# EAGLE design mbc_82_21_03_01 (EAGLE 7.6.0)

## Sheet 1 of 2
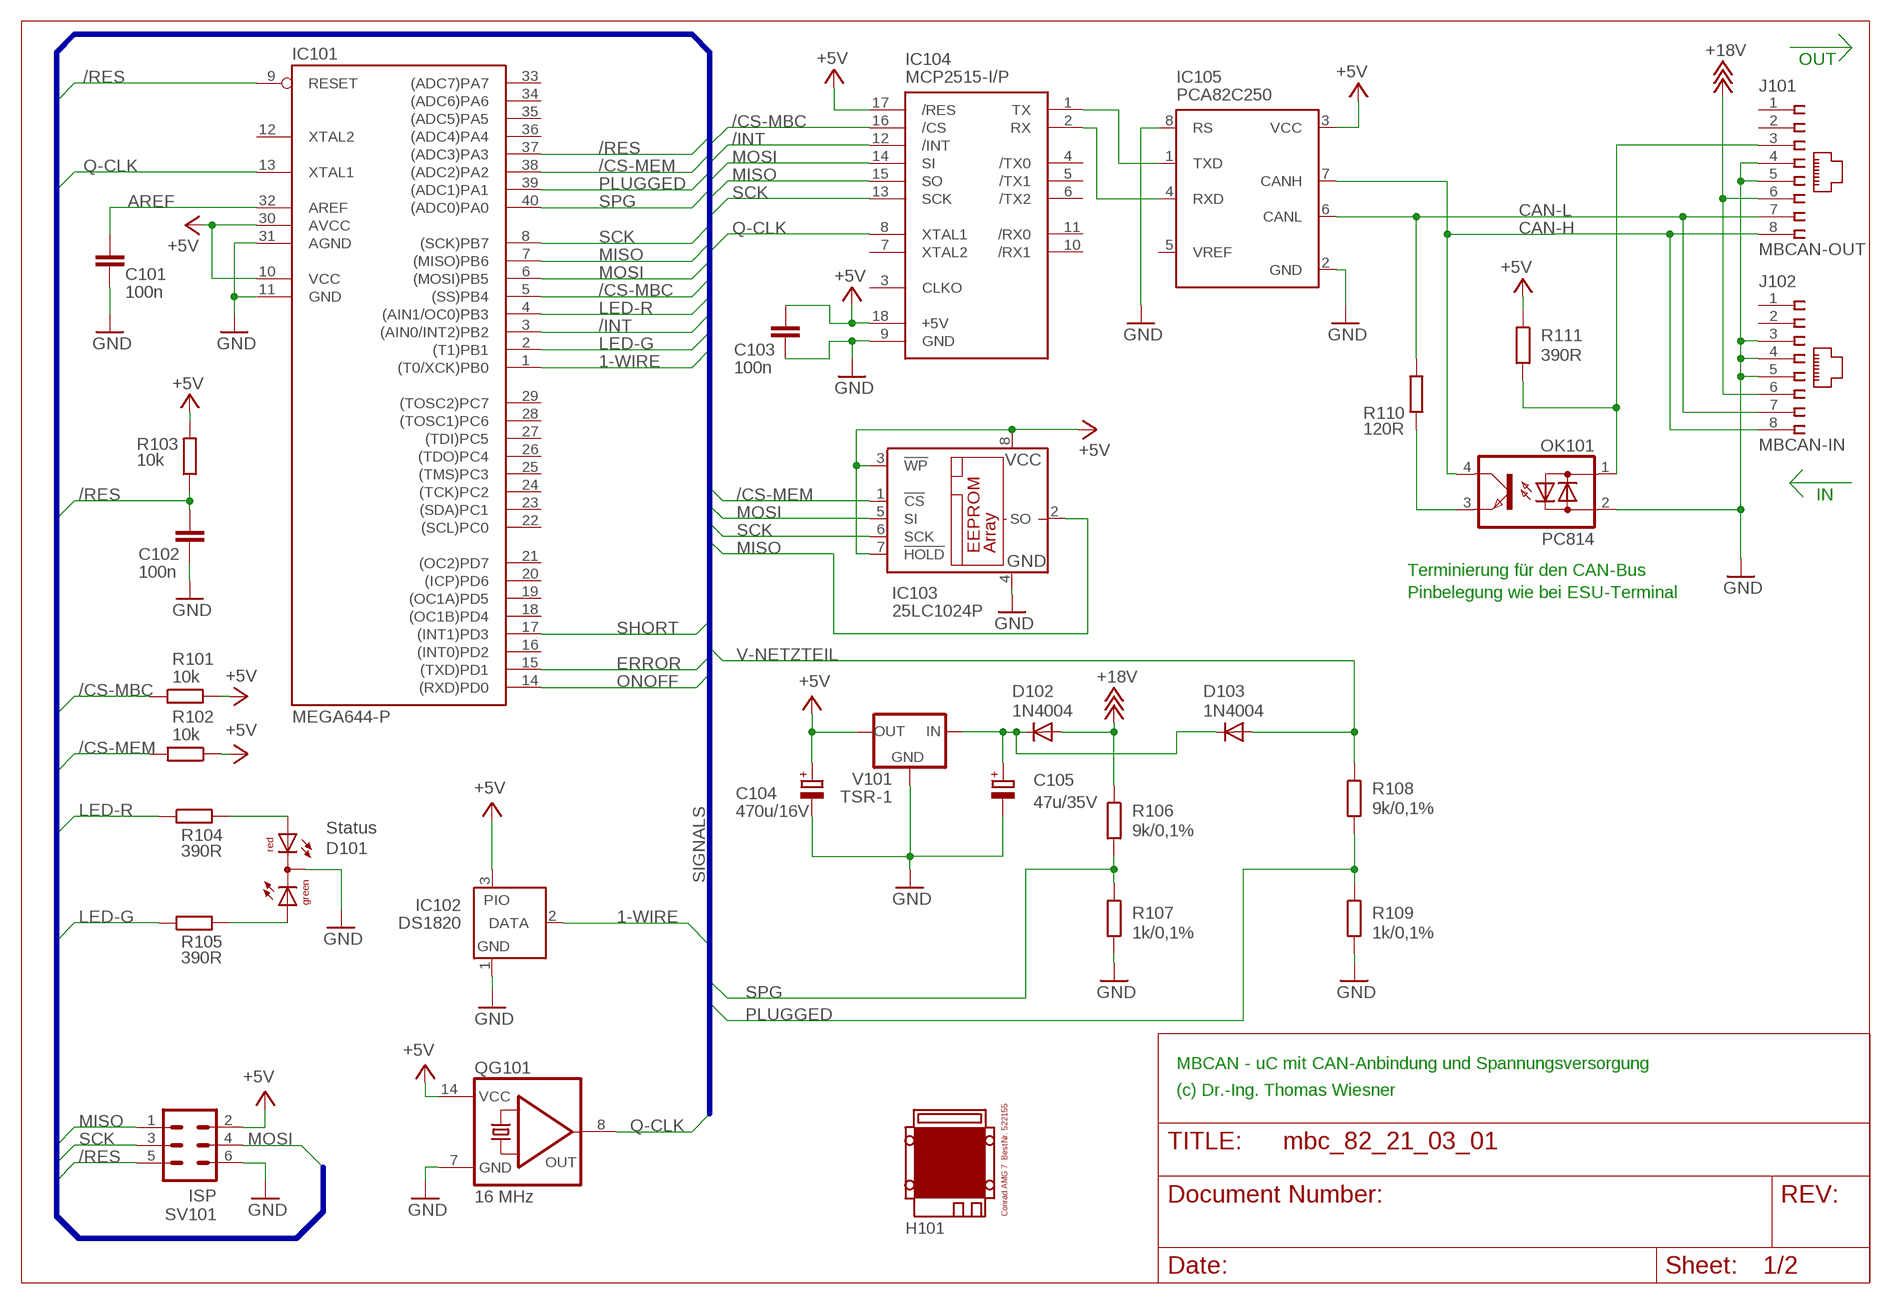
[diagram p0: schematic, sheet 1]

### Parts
C101  100n  C-EU025-025X050  [C025-025X050]
C102  100n  C-EU025-025X050  [C025-025X050]
C103  100n  C-EU025-025X050  [C025-025X050]
C104  470u/16V  CPOL-EUE3.5-8  [E3,5-8]
C105  47u/35V  CPOL-EUE2.5-7  [E2,5-7]
D101  Status  DUOLED5MM  [DUOLED5MM]
D102  1N4004  [DO41-10]
D103  1N4004  [DO41-10]
H101  MODULGEHÄUSE-AMG-7  [MODULGEHÄUSE-AMG-7]
IC101  MEGA644-P  MEGA323-P  [DIL40]
IC102  DS1820  DS2405  [TO92-]
IC103  25LC1024P  25LC040P  [DIL8]
IC104  MCP2515-I/P  MCP2510-I/P  [DIL18]
IC105  PCA82C250  [DIL08]
J101  MBCAN-OUT  215877-4  [215877-4]
J102  MBCAN-IN  215877-4  [215877-4]
OK101  PC814  [DIL04]
QG101  16 MHz  QG5860  [DIL14S]
R101  10k  R-EU_0207/10  [0207/10]
R102  10k  R-EU_0207/10  [0207/10]
R103  10k  R-EU_0207/10  [0207/10]
R104  390R  R-EU_0207/10  [0207/10]
R105  390R  R-EU_0207/10  [0207/10]
R106  9k/0,1%  R-EU_0207/10  [0207/10]
R107  1k/0,1%  R-EU_0207/10  [0207/10]
R108  9k/0,1%  R-EU_0207/10  [0207/10]
R109  1k/0,1%  R-EU_0207/10  [0207/10]
R110  120R  R-EU_0207/10  [0207/10]
R111  390R  R-EU_0207/10  [0207/10]
SV101  ISP  ML6  [ML6]
V101  TSR-1  [TRACO-TSR-1]

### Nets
1-WIRE: IC101.1((T0/XCK)PB0) IC102.2(DATA)
+5V: C103.1 C104.+ IC101.10(VCC) IC101.30(AVCC) IC102.3(PIO) IC103.3(!WP) IC103.7(!HOLD) IC103.8(VCC) IC104.17(/RES) IC104.18(+5V) IC105.3(VCC) QG101.14(VCC) R101.2 R102.1 R103.2 R111.1 SV101.2 V101.OUT ; also sheet 2
+18V: D102.A J101.6 J102.6 R106.1
/CS-MBC: IC101.5((SS)PB4) IC104.16(/CS) R101.1
/CS-MEM: IC101.38((ADC2)PA2) IC103.1(!CS) R102.2
/INT: IC101.3((AIN0/INT2)PB2) IC104.12(/INT)
/RES: C102.1 IC101.9(RESET) IC101.37((ADC3)PA3) R103.1 SV101.5
AREF: C101.1 IC101.32(AREF)
CAN-H: IC105.7(CANH) J101.8 J102.8 OK101.4(C)
CAN-L: IC105.6(CANL) J101.7 J102.7 R110.2
ERROR: IC101.15((TXD)PD1) ; also sheet 2
GND: C101.2 C102.2 C103.2 C104.- C105.- D101.K(C) IC101.11(GND) IC101.31(AGND) IC102.1(GND) IC103.4(GND) IC104.9(GND) IC105.2(GND) IC105.8(RS) J101.4 J101.5 J102.3 J102.4 J102.5 OK101.2(AC2) QG101.7(GND) R107.2 R109.2 SV101.6 V101.GND ; also sheet 2
LED-G: IC101.2((T1)PB1) R105.1
LED-R: IC101.4((AIN1/OC0)PB3) R104.1
MISO: IC101.7((MISO)PB6) IC103.2(SO) IC104.15(SO) SV101.1
MOSI: IC101.6((MOSI)PB5) IC103.5(SI) IC104.14(SI) SV101.4
N$1: IC104.1(TX) IC105.1(TXD)
N$2: IC104.2(RX) IC105.4(RXD)
N$3: OK101.3(E) R110.1
N$4: J101.3 OK101.1(AC1) R111.2
N$6: C105.+ D102.C D103.C V101.IN
N$9: D101.AR R104.2
N$13: D101.AG R105.2
ONOFF: IC101.14((RXD)PD0) ; also sheet 2
PLUGGED: IC101.39((ADC1)PA1) R108.2 R109.1
Q-CLK: IC101.13(XTAL1) IC104.8(XTAL1) QG101.8(OUT)
SCK: IC101.8((SCK)PB7) IC103.6(SCK) IC104.13(SCK) SV101.3
SHORT: IC101.17((INT1)PD3) ; also sheet 2
SPG: IC101.40((ADC0)PA0) R106.2 R107.1
V-NETZTEIL: D103.A R108.1 ; also sheet 2
Unconnected: IC101.12(XTAL2) IC101.16((INT0)PD2) IC101.18((OC1B)PD4) IC101.19((OC1A)PD5) IC101.20((ICP)PD6) IC101.21((OC2)PD7) IC101.22((SCL)PC0) IC101.23((SDA)PC1) IC101.24((TCK)PC2) IC101.25((TMS)PC3) IC101.26((TDO)PC4) IC101.27((TDI)PC5) IC101.28((TOSC1)PC6) IC101.29((TOSC2)PC7) IC101.33((ADC7)PA7) IC101.34((ADC6)PA6) IC101.35((ADC5)PA5) IC101.36((ADC4)PA4) IC104.3(CLKO) IC104.4(/TX0) IC104.5(/TX1) IC104.6(/TX2) IC104.7(XTAL2) IC104.10(/RX1) IC104.11(/RX0) IC105.5(VREF) J101.1 J101.2 J102.1 J102.2

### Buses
SIGNALS

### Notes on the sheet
- OUT
- IN
- Terminierung für den CAN-Bus
- Pinbelegung wie bei ESU-Terminal
- MBCAN - uC mit CAN-Anbindung und Spannungsversorgung
- (c) Dr.-Ing. Thomas Wiesner

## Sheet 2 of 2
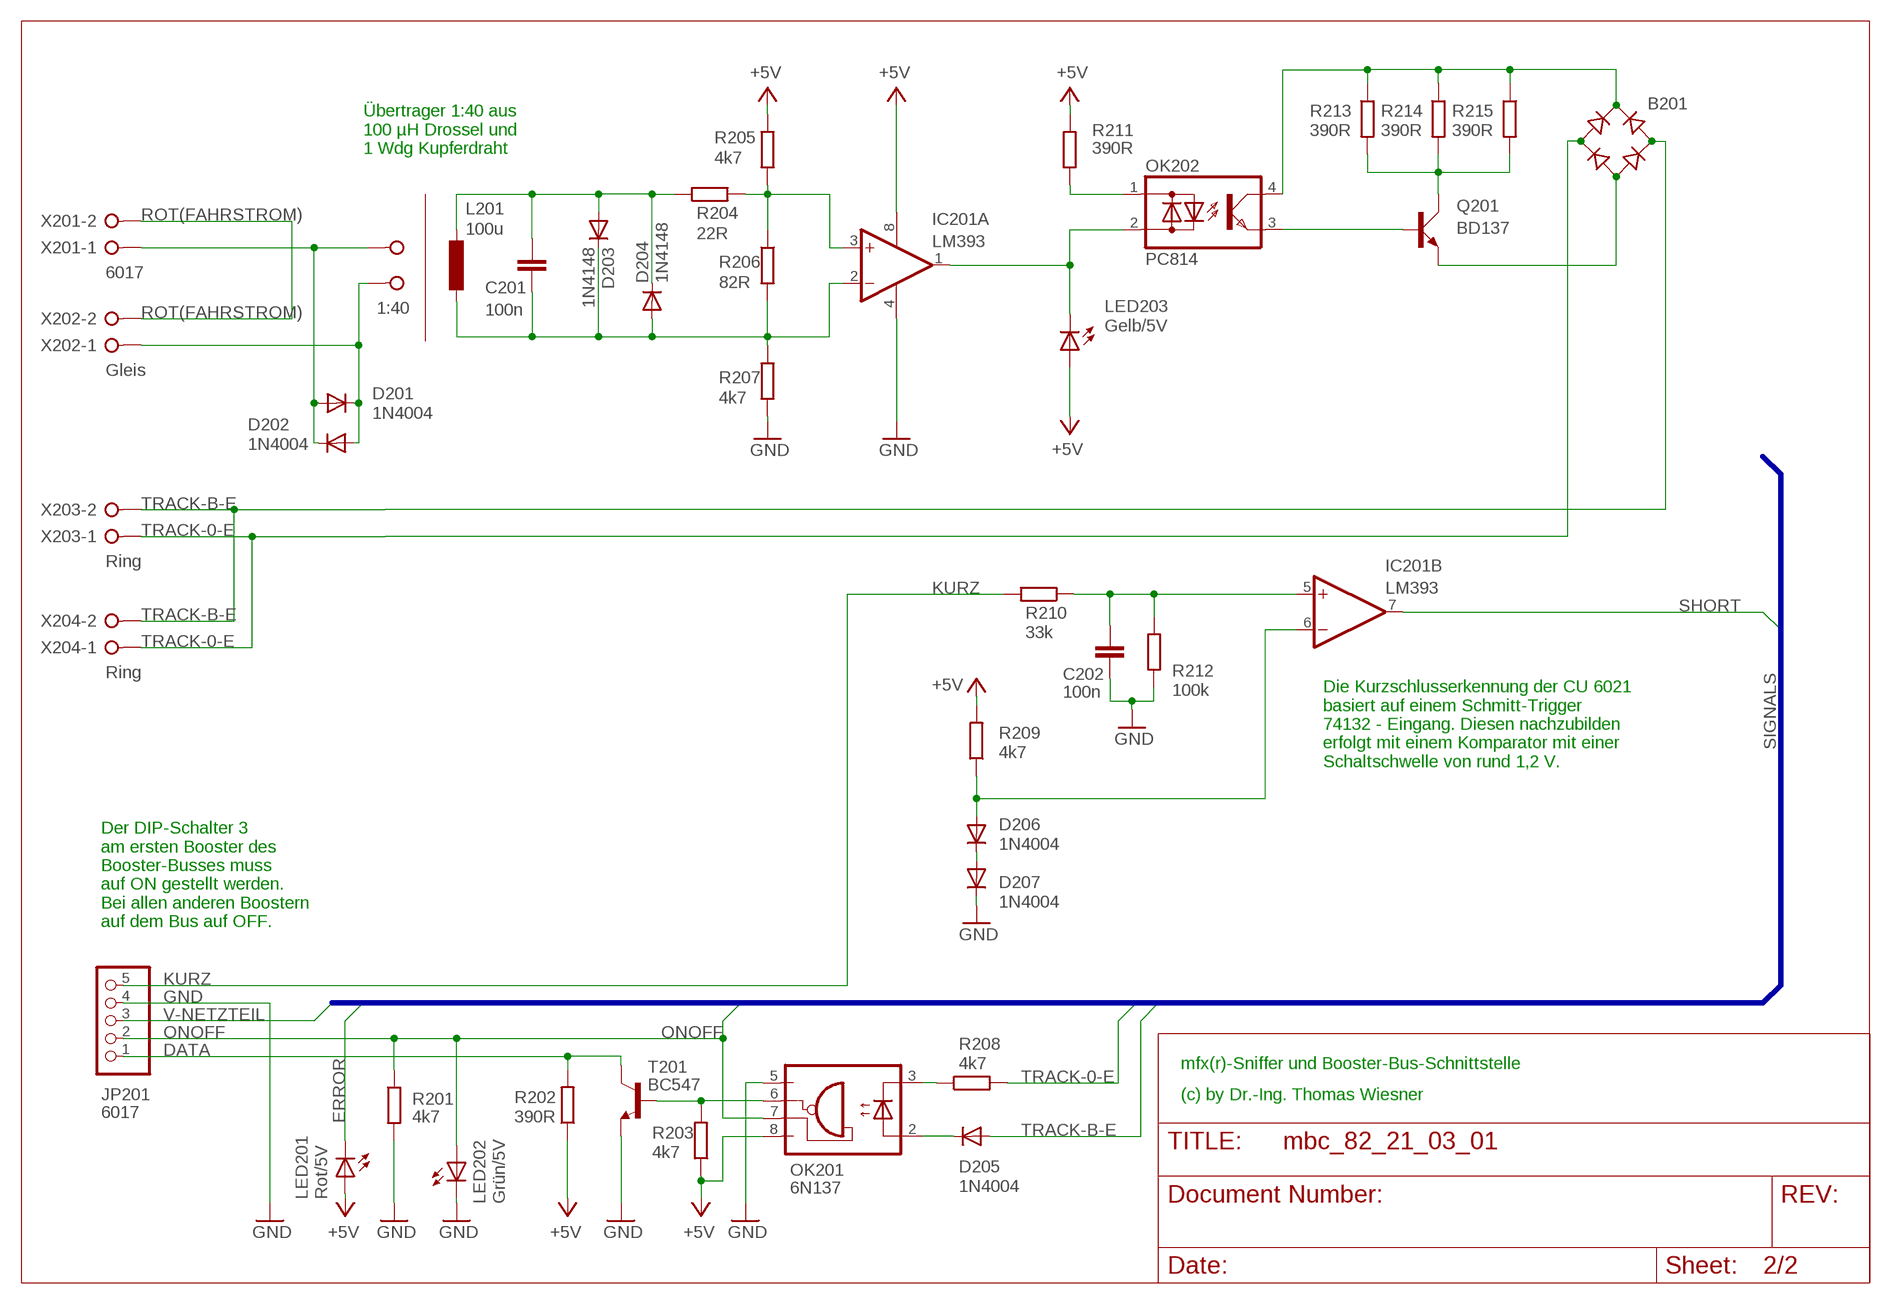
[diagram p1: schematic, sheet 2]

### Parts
B201  RB1A  [RB1A]
C201  100n  C-EU025-025X050  [C025-025X050]
C202  100n  C-EU025-025X050  [C025-025X050]
D201  1N4004  [DO41-10]
D202  1N4004  [DO41-10]
D203  1N4148  1N4148DO35-10  [DO35-10]
D204  1N4148  1N4148DO35-10  [DO35-10]
D205  1N4004  [DO41-10]
D206  1N4004  [DO41-10]
D207  1N4004  [DO41-10]
IC201  LM393  [DIL08]
JP201  6017  PINHD-1X5  [1X05]
L201  100u  L-EU6000-XXX-RC  [6000-XXXX-RC]
LED201  Rot/5V  LED3MM  [LED3MM]
LED202  Grün/5V  LED3MM  [LED3MM]
LED203  Gelb/5V  LED3MM  [LED3MM]
OK201  6N137  [DIL08]
OK202  PC814  [DIL04]
Q201  BD137  BD139  [TO126AV]
R201  4k7  R-EU_0207/10  [0207/10]
R202  390R  R-EU_0207/10  [0207/10]
R203  4k7  R-EU_0207/10  [0207/10]
R204  22R  R-EU_0207/10  [0207/10]
R205  4k7  R-EU_0207/10  [0207/10]
R206  82R  R-EU_0207/10  [0207/10]
R207  4k7  R-EU_0207/10  [0207/10]
R208  4k7  R-EU_0207/10  [0207/10]
R209  4k7  R-EU_0207/10  [0207/10]
R210  33k  R-EU_0207/10  [0207/10]
R211  390R  R-EU_0207/10  [0207/10]
R212  100k  R-EU_0207/10  [0207/10]
R213  390R  R-EU_0207/10  [0207/10]
R214  390R  R-EU_0207/10  [0207/10]
R215  390R  R-EU_0207/10  [0207/10]
T201  BC547  [TO92]
TP  1:40  W237-02P  [W237-132]
X201  6017  W237-02P  [W237-132]
X202  Gleis  W237-02P  [W237-132]
X203  Ring  W237-02P  [W237-132]
X204  Ring  W237-02P  [W237-132]

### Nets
+5V: IC201.8(A:V+) LED201.A LED203.A OK201.8(VCC) R202.1 R203.1 R205.2 R209.2 R211.2 ; also sheet 1
DATA: JP201.1 R202.2 T201.3(C)
ERROR: LED201.K(C) ; also sheet 1
GND: C202.2 D207.C IC201.4(A:V-) JP201.4 LED202.K(C) OK201.5(GND) R201.2 R207.2 R212.2 T201.1(E) ; also sheet 1
KURZ: JP201.5 R210.2
N$5: OK202.3(E) Q201.B
N$7: D205.C OK201.2(A)
N$8: OK201.3(C) R208.1
N$12: B201.- Q201.E
N$14: C201.2 D203.C D204.A IC201.2(A:-IN) L201.2 R206.2 R207.1
N$15: IC201.3(A:+IN) R204.2 R205.1 R206.1
N$16: D201.C D202.A TP.1 X202.1
N$17: B201.+ OK202.4(C) R213.1 R214.1 R215.1
N$18: Q201.C R213.2 R214.2 R215.2
N$19: C201.1 D203.A D204.C L201.1 R204.1
N$20: D206.C D207.A
N$21: OK202.1(AC1) R211.1
N$22: IC201.1(A:COLOUT) LED203.K(C) OK202.2(AC2)
N$23: D206.A IC201.6(B:-IN) R209.1
N$24: C202.1 IC201.5(B:+IN) R210.1 R212.1
N$29: OK201.6(VO) R203.2 T201.2(B)
O': D201.A D202.C TP.2 X201.1
ONOFF: JP201.2 LED202.A OK201.7(VE) R201.1 ; also sheet 1
ROT(FAHRSTROM): X201.2 X202.2
SHORT: IC201.7(B:COLOUT) ; also sheet 1
TRACK-0-E: B201.AC1 R208.2 X203.1 X204.1
TRACK-B-E: B201.AC2 D205.A X203.2 X204.2
V-NETZTEIL: JP201.3 ; also sheet 1

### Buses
SIGNALS

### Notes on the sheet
- Übertrager 1:40 aus
  100 µH Drossel und 
  1 Wdg Kupferdraht
- Die Kurzschlusserkennung der CU 6021
  basiert auf einem Schmitt-Trigger 
  74132 - Eingang. Diesen nachzubilden 
  erfolgt mit einem Komparator mit einer
  Schaltschwelle von rund 1,2 V.
- Der DIP-Schalter 3
  am ersten Booster des
  Booster-Busses muss
  auf ON gestellt werden.
  Bei allen anderen Boostern
  auf dem Bus auf OFF.
- mfx(r)-Sniffer und Booster-Bus-Schnittstelle
- (c) by Dr.-Ing. Thomas Wiesner

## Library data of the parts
B201 = rectifier:RB1A: RECTIFIER 1 A
C101-C103 C201 C202 = rcl:C-EU: CAPACITOR, European symbol
C104 C105 = rcl:CPOL-EU: POLARIZED CAPACITOR, European symbol
D101 = led:DUOLED5MM: DUO LED 2 colors, 5 mm, round
D102 D103 D201 D202 D205-D207 = diode:1N4004: DIODE
D203 D204 = diode:1N4148: DIODE
H101 = mbc:MODULGEHÄUSE-AMG-7: Gehäuse
IC101 = atmel:MEGA323-P: MICROCONTROLLER 32 Kbytes FLASH 2 Kbytes SRAM 1 Kbytes EEPROM USART 8-channel 10 bit ADC Source: avr.lbr; OC_FARNELL: unknown; OC_NEWARK: unknown
IC102 = maxim:DS2405: Addressable Switch DALLAS Semiconductor; MF: DALLAS SEMICONDUCTOR; MPN: DS2405; OC_FARNELL: 1188025; OC_NEWARK: 06F4645
IC103 = microchip:25*: Serial EEPROM 4K/ 8K , SPI bus; MF: MICROCHIP; MPN: 25LC040/P; OC_FARNELL: 9758100; OC_NEWARK: 96K4091
IC104 = mbc:MCP2510: BASIC-CAN 2.0a Controller Stand-alone CAN controller von Microchip
IC105 = micro-philips:PCA82C250: CAN CONTROLLER INTERFACE; OC_FARNELL: 3692358; OC_NEWARK: unknown
IC201 = mbc:LM393: DC-Comparator Dual
J101 J102 = con-amp:215877-4: AMP connector
JP201 = pinhead:PINHD-1X5: PIN HEADER
L201 = rcl:L-EU: INDUCTOR, European symbol
LED201-LED203 = led:LED: LED
OK101 OK202 = optocoupler:PC814: SHARP OPTO COUPLER; OC_FARNELL: 9707662; OC_NEWARK: unknown
OK201 = optocoupler:6N137: MOTOROLA OPTO COUPLER; MPN: 6N137; OC_FARNELL: 1328376; OC_NEWARK: 52M1895
Q201 = transistor-power:BD139: NPN TRANSISTOR
QG101 = crystal:QG5860: CRYSTAL RESONATOR; OC_FARNELL: unknown; OC_NEWARK: unknown
R101-R111 R201-R215 = resistor:R-EU_: RESISTOR, European symbol
SV101 = con-ml:ML6: HARTING; OC_FARNELL: unknown; OC_NEWARK: unknown
T201 = transistor:BC547: NPN TRANSISTOR
TP X201-X204 = con-wago-508:W237-02P: WAGO SREW CLAMP; OC_FARNELL: unknown; OC_NEWARK: unknown
V101 = mbc:TSR-1: Spannungsregler Hersteller: TRACO Typ: TSR-1 5V: TSR 1-2450 Spg: 5V Strom: 1A Reichelt TSR 1-2450

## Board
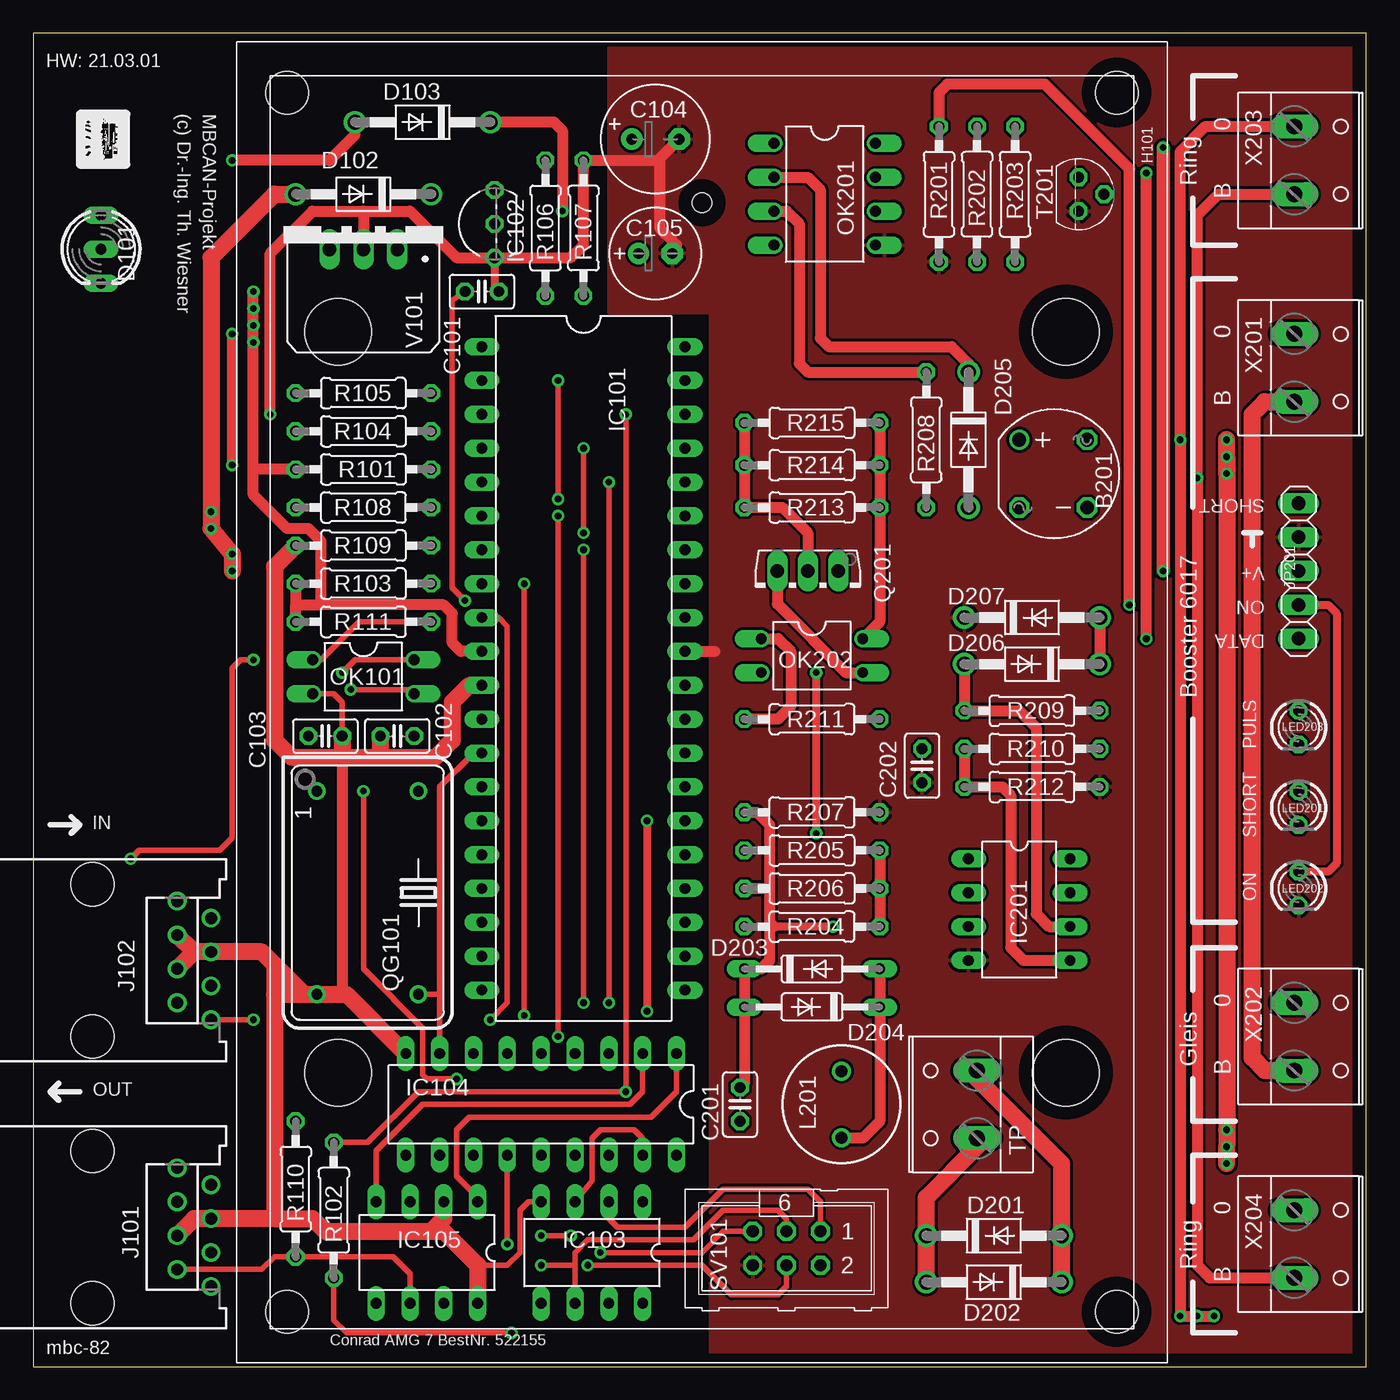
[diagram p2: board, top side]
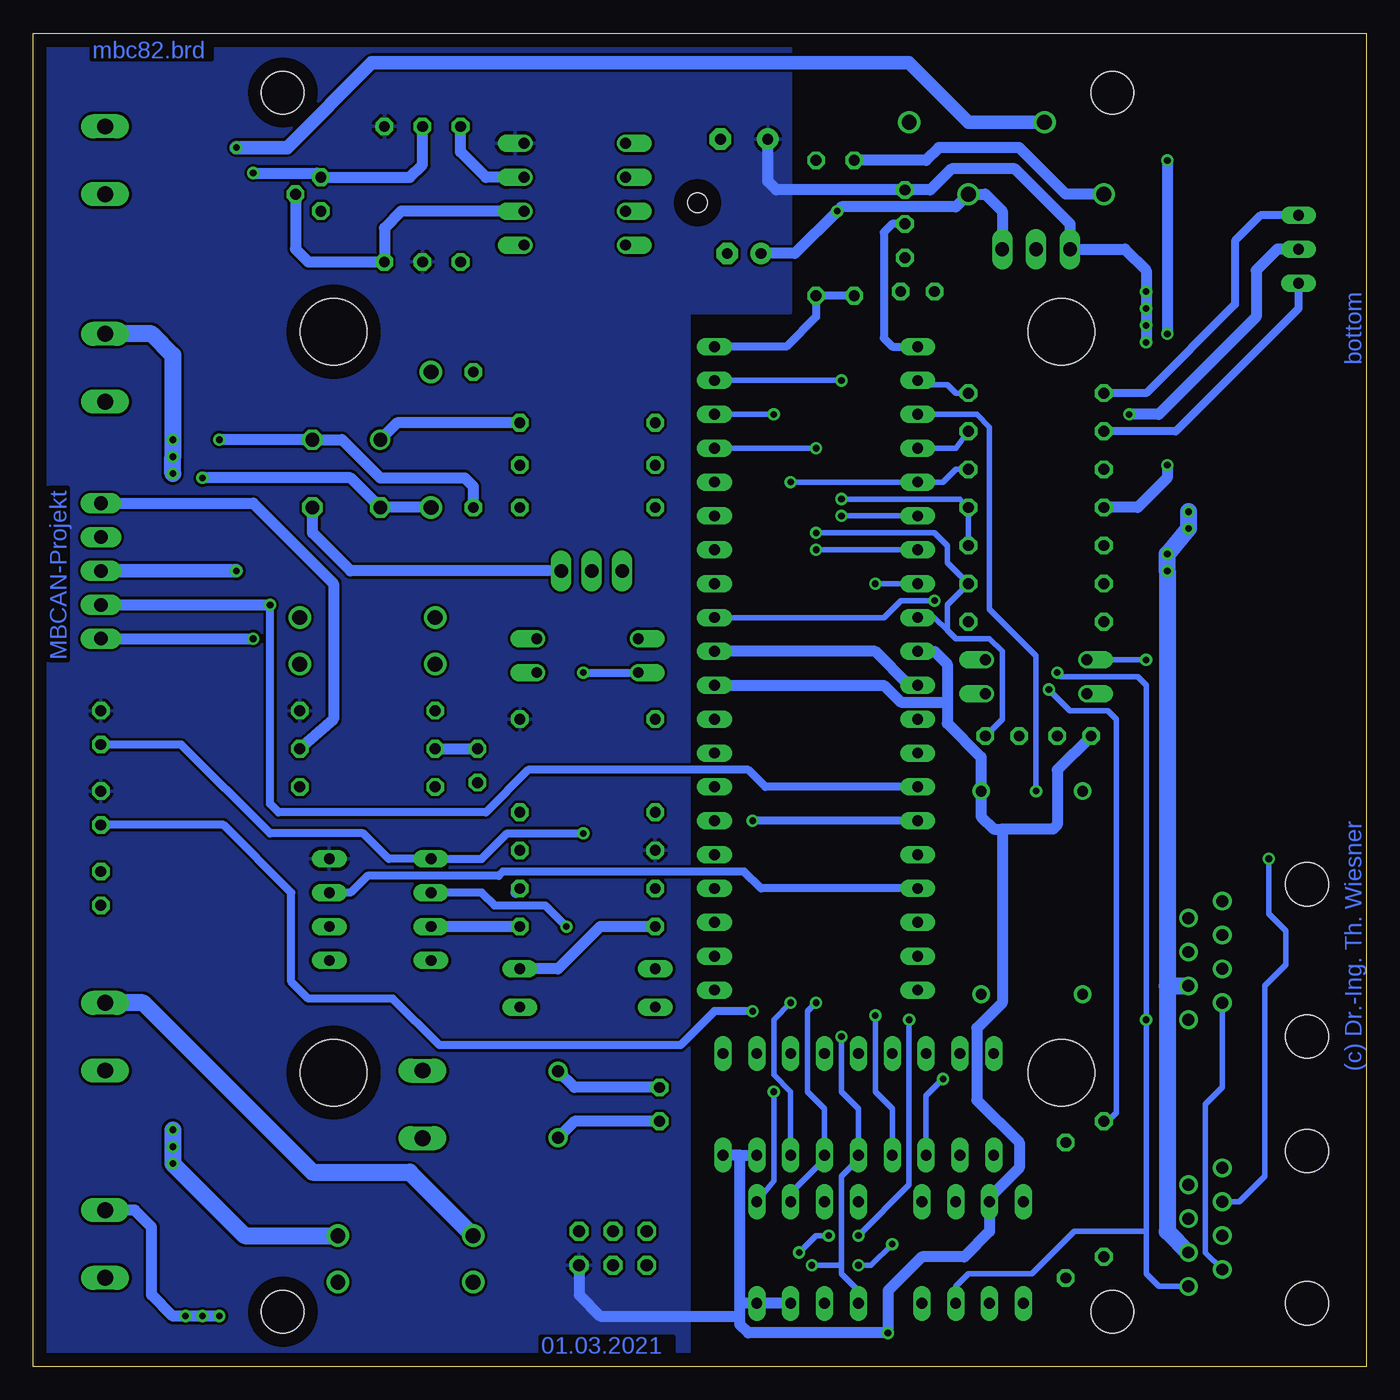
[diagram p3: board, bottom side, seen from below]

Size 100 x 99.99 mm. Coordinates in mm from the lower left corner, seen from the top.
Outline: 0,99.99 0,0 100,0 100,99.99 0,99.99
Copper layers (1*16): Top 0.035mm / dielectric 1.5mm / Bottom 0.035mm
Design rules "default *": minimum track width 10mil, minimum drill 0.5mm, track to track 8mil, track to pad 8mil, pad to pad 8mil, via to via 8mil, smd to smd 8mil, copper to edge 40mil, drill to drill 8mil, minimum pad ring 10mil, minimum via ring 8mil, stop-mask expansion 4mil, vias tented up to drill 0mil, thermal gap 10mil

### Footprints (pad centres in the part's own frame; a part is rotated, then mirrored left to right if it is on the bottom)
RB1A = drill 1.016: + -2.54,2.54 | drill 1.016 octagon: - 2.54,-2.54; AC1 2.54,2.54; AC2 -2.54,-2.54
C025-025X050 = drill 0.813 octagon: 1 -1.27,0; 2 1.27,0
E3,5-8 = drill 0.813 pad 1.6: + -1.778,0 | drill 0.813 pad 1.6 octagon: - 1.778,0
E2,5-7 = drill 0.813 pad 1.6: + -1.27,0 | drill 0.813 pad 1.6 octagon: - 1.27,0
DUOLED5MM = drill 0.813 long: AG -2.54,0; AR 2.54,0; K 0,0
DO41-10 = drill 1.118: A 5.08,0; C -5.08,0
DO35-10 = drill 0.813 long: A 5.08,0; C -5.08,0
MODULGEHÄUSE-AMG-7 = hole 3.2: -45.72,-31.115; -45.72,31.115; 45.72,31.115; 45.72,-31.115 | hole 5: -27.781,-27.305; 27.781,-27.305; -27.781,27.305; 27.781,27.305 | hole 1.5: -37.465,0
DIL40 = drill 0.813 long: 1 -24.13,-7.62; 2 -21.59,-7.62; 3 -19.05,-7.62; 4 -16.51,-7.62; 5 -13.97,-7.62; 6 -11.43,-7.62; 7 -8.89,-7.62; 8 -6.35,-7.62; 9 -3.81,-7.62; 10 -1.27,-7.62; 11 1.27,-7.62; 12 3.81,-7.62; 13 6.35,-7.62; 14 8.89,-7.62; 15 11.43,-7.62; 16 13.97,-7.62; 17 16.51,-7.62; 18 19.05,-7.62; 19 21.59,-7.62; 20 24.13,-7.62; 21 24.13,7.62; 22 21.59,7.62; 23 19.05,7.62; 24 16.51,7.62; 25 13.97,7.62; 26 11.43,7.62; 27 8.89,7.62; 28 6.35,7.62; 29 3.81,7.62; 30 1.27,7.62; 31 -1.27,7.62; 32 -3.81,7.62; 33 -6.35,7.62; 34 -8.89,7.62; 35 -11.43,7.62; 36 -13.97,7.62; 37 -16.51,7.62; 38 -19.05,7.62; 39 -21.59,7.62; 40 -24.13,7.62
TO92- = drill 0.813 octagon: 1 -2.54,0; 2 0,0; 3 2.54,0
DIL8 = drill 0.813 long: 1 -3.81,-3.81; 2 -1.27,-3.81; 3 1.27,-3.81; 4 3.81,-3.81; 5 3.81,3.81; 6 1.27,3.81; 7 -1.27,3.81; 8 -3.81,3.81
DIL18 = drill 0.813 long: 1 -10.16,-3.81; 2 -7.62,-3.81; 3 -5.08,-3.81; 4 -2.54,-3.81 | drill 0.8 long: 5 0,-3.81; 6 2.54,-3.81; 7 5.08,-3.81; 8 7.62,-3.81; 9 10.16,-3.81; 10 10.16,3.81; 11 7.62,3.81; 12 5.08,3.81; 13 2.54,3.81; 14 0,3.81; 15 -2.54,3.81; 16 -5.08,3.81; 17 -7.62,3.81; 18 -10.16,3.81
DIL08 = drill 0.813 long: 1 -3.81,-3.81; 2 -1.27,-3.81; 3 1.27,-3.81; 4 3.81,-3.81; 5 3.81,3.81; 6 1.27,3.81; 7 -1.27,3.81; 8 -3.81,3.81
215877-4 = drill 0.889: 1 -4.445,6.35; 2 -3.175,8.89; 3 -1.905,6.35; 4 -0.635,8.89; 5 0.635,6.35; 6 1.905,8.89; 7 3.175,6.35; 8 4.445,8.89 | hole 3.251: -5.715,0; 5.715,0
1X05 = drill 1.016 long: 1 -5.08,0; 2 -2.54,0; 3 0,0; 4 2.54,0; 5 5.08,0
6000-XXXX-RC = drill 0.9 pad 1.422: 1 -2.5,0; 2 2.5,0
LED3MM = drill 0.813 octagon: A -1.27,0; K 1.27,0
DIL04 = drill 0.813 offset: 1 -1.27,-3.81; 2 1.27,-3.81; 3 1.27,3.81; 4 -1.27,3.81
DIL08' = drill 0.813 offset: 1 -3.81,-3.81; 2 -1.27,-3.81; 3 1.27,-3.81; 4 3.81,-3.81; 5 3.81,3.81; 6 1.27,3.81; 7 -1.27,3.81; 8 -3.81,3.81
TO126AV = drill 1.016 long: B 2.286,-1.27; C 0,-1.27; E -2.286,-1.27
DIL14S = drill 0.813: 1 -7.62,-3.81; 7 7.62,-3.81; 8 7.62,3.81; 14 -7.62,3.81
0207/10 = drill 0.813 octagon: 1 -5.08,0; 2 5.08,0
ML6 = drill 0.914 octagon: 1 -2.54,-1.27; 2 -2.54,1.27; 3 0,-1.27; 4 0,1.27; 5 2.54,-1.27; 6 2.54,1.27
TO92 = drill 0.813 octagon: 1 1.27,0; 2 0,1.905; 3 -1.27,0
W237-132 = drill 1.194 long: 1 -2.54,-0.635; 2 2.54,-0.635
TRACO-TSR-1 = drill 1.016 long: GND 0,2.54; IN -2.54,2.54; OUT 2.54,2.54

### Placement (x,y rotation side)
B201  76.52,66.97 0 top
C101  33.66,80.62 0 top
C102  27.3,47.29 180 top
C103  21.91,47.29 0 top
C104  46.67,92.06 0 top
C105  46.67,83.48 0 top
C201  53.02,19.66 90 top
C202  66.67,45.06 270 top
D101  5.08,83.8 270 top
D102  24.77,87.93 180 top
D103  29.21,93.33 180 top
D201  72.07,9.82 0 top
D202  72.07,6.33 180 top
D203  58.42,29.82 0 top
D204  58.42,26.97 180 top
D205  70.17,69.51 270 top
D206  74.93,52.68 180 top
D207  74.93,56.18 0 top
H101  50.16,49.83 270 top
IC101  41.27,52.37 270 top
IC102  34.61,85.7 90 top
IC103  41.91,8.55 180 top
IC104  38.1,19.66 180 top
IC105  29.53,8.55 180 top
IC201  73.98,34.27 270 top
J101  4.45,10.46 270 top
J102  4.45,30.46 270 top
JP201  94.93,59.67 90 top
L201  60.64,19.66 90 top
LED201  94.93,41.89 270 top
LED202  94.93,35.86 270 top
LED203  94.93,47.92 270 top
OK101  24.77,51.73 270 top
OK201  6N137  [DIL08']  59.37,87.93 270 top
OK202  58.42,53.32 270 top
Q201  58.1,58.4 180 top
QG101  25.08,35.54 270 top
R101  24.77,67.29 180 top
R102  22.54,11.73 90 top
R103  24.77,58.72 180 top
R104  24.77,70.15 180 top
R105  24.77,73.01 180 top
R106  38.42,85.39 270 top
R107  41.27,85.39 90 top
R108  24.77,64.43 0 top
R109  24.77,61.57 180 top
R110  19.68,13.32 270 top
R111  24.77,55.86 0 top
R201  67.94,87.93 270 top
R202  70.8,87.93 90 top
R203  73.66,87.93 270 top
R204  58.42,33 0 top
R205  58.42,38.71 180 top
R206  58.42,35.86 180 top
R207  58.42,41.57 0 top
R208  66.99,69.51 270 top
R209  74.93,49.19 0 top
R210  74.93,46.33 0 top
R211  58.42,48.56 0 top
R212  74.93,43.48 0 top
R213  58.42,64.43 180 top
R214  58.42,67.61 180 top
R215  58.42,70.78 180 top
SV101  56.52,8.87 180 top
T201  78.42,87.93 270 top
TP  70.17,19.66 90 top
V101  24.77,86.34 180 top
X201  95.25,74.91 270 top
X202  95.25,24.75 270 top
X203  95.25,90.47 270 top
X204  95.25,9.19 270 top

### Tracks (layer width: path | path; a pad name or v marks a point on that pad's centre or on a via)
1-WIRE
  Bottom 0.61: IC102.2 35.56,85.7 36.2,85.07 36.2,77.13 35.56,76.5 IC101.1
+5V  (via drill 0.5)
  Top 0.406: R102.1 22.54,3.47 23.5,2.52 v35.88,2.52 | IC103.3 41.91,13.95 41.91,17.12 42.55,17.76 45.09,17.76 45.72,17.12 IC104.17
  Top 0.813: IC101.10 32.07,53.64 31.43,54.27 31.43,56.49 30.8,57.13 21.59,57.13 | 21.59,57.13 21.59,61.89 20.64,62.84 19.05,62.84 16.51,65.39 16.51,67.29 | 16.51,67.29 v16.51,76.81 v16.51,78.09 v16.51,79.36 v16.51,80.62 | R103.2 19.68,57.13 | R111.1 19.68,57.13 | 19.68,57.13 21.59,57.13 | R101.2 16.51,67.29
  Bottom 0.406: C104.+ 44.9,89.83
  Bottom 0.813: v16.51,76.81 v16.51,78.09 v16.51,79.36 v16.51,80.62 16.51,82.21 18.1,83.8 V101.OUT 22.23,85.7 26.35,89.83 31.11,89.83 32.7,88.25 IC102.3 44.26,88.25 44.9,88.88 C104.+ | 46.99,15.86 IC104.18 | 46.99,15.86 IC104.17 | 46.99,4.74 46.99,15.86 | 46.99,3.79 46.99,3.15 46.35,2.52 v35.88,2.52 35.88,5.7 33.34,8.24 30.16,8.24 28.26,10.14 IC105.3 28.26,12.68 26.04,14.9 26.04,16.81 29.21,19.98 29.21,25.38 27.3,27.29 27.3,40.3 | 46.99,3.79 46.99,4.74 | IC101.10 32.38,53.64 31.43,52.68 31.43,49.83 | 27.3,40.3 27.94,40.3 28.89,41.25 QG101.14 28.89,45.7 31.43,48.24 31.43,49.83 | C103.1 23.18,44.75 23.18,40.62 23.5,40.3 27.3,40.3 | IC103.7 IC103.8 46.99,4.74 | IC101.30 36.2,51.1 34.92,49.83 31.43,49.83 | SV101.2 59.05,5.38 57.47,3.79 46.99,3.79
  pour Bottom: 43.18,99.67 43.18,79.04 50.8,79.04 50.8,0.3 99.69,0.3 99.69,99.67
+18V  (via drill 0.5)
  Top 1.27: D102.A 18.1,87.93 13.34,83.17 v13.34,62.84 v14.92,60.94 v14.92,59.67
  Bottom 0.813: R106.1 33.02,90.47 32.07,91.42 26.04,91.42 22.54,87.93 D102.A
  Bottom 1.27: 14.92,28.55 v14.92,59.67 v14.92,60.94 v13.34,62.84 v13.34,64.12 | 14.92,28.55 J102.6 | 14.92,28.55 14.92,10.14 J101.6
/CS-MBC  (via drill 0.5)
  Top 0.406: v43.18,66.34 v43.18,27.29
  Bottom 0.406: v43.18,66.34 IC101.5 31.75,66.34 30.8,67.29 R101.1 | v43.18,27.29 44.45,26.02 44.45,21.89 43.18,20.62 IC104.16
/CS-MEM  (via drill 0.5)
  Top 0.406: v44.45,71.42 v44.45,20.62 28.89,20.62 25.08,16.81 R102.2
  Bottom 0.406: v44.45,20.62 44.45,13.95 IC103.1 | v44.45,71.42 IC101.38
/INT  (via drill 0.5)
  Top 0.406: v31.75,21.57 29.53,21.57 29.21,21.89 29.21,25.38 24.77,29.82 v24.77,43.16
  Bottom 0.406: IC104.12 33.02,20.3 v31.75,21.57 | v24.77,43.16 24.77,53.32 28.26,56.81 28.26,70.47 29.21,71.42 IC101.3
/RES  (via drill 0.5)
  Top 0.406: v34.29,26.02 35.56,27.29 35.56,55.54 34.92,56.18 IC101.9 | v41.27,68.88 v41.27,62.53 | v38.1,9.82 v40.32,9.82 | v42.55,8.55 50.16,8.55 51.75,10.14 SV101.5
  Bottom 0.406: v38.1,9.82 34.29,13.63 v34.29,26.02 | IC101.9 32.38,56.18 31.43,55.22 | C102.1 27.3,48.56 27.3,53.64 28.26,54.59 30.8,54.59 31.43,55.22 | 31.43,55.22 31.43,57.13 R103.1 31.43,60.3 31.43,61.57 32.38,62.53 v41.27,62.53 | IC101.37 v41.27,68.88 | v40.32,9.82 41.27,9.82 v42.55,8.55
AREF  (via drill 0.5)
  Top 0.406: v32.38,57.45 31.43,58.4 31.43,79.99 C101.1
  Bottom 0.406: IC101.32 36.2,56.18 34.92,57.45 v32.38,57.45
CAN-H  (via drill 0.5)
  Top 0.406: v16.51,26.02 J102.8 | OK101.4 24.13,53 v23.18,52.05
  Bottom 0.406: 16.51,10.14 v16.51,26.02 16.51,51.1 17.14,51.73 22.86,51.73 v23.18,52.05 | J101.8 15.56,6.01 16.51,6.97 16.51,10.14 | IC105.7 30.8,6.01 29.84,6.97 25.08,6.97 21.91,10.14 16.51,10.14
CAN-L
  Top 0.406: J101.7 17.14,7.28 18.1,8.24 R110.2 26.99,8.24 28.26,6.97 IC105.6
  Bottom 0.406: J101.7 12.06,8.55 12.06,19.66 10.79,20.93 J102.7
DATA  (via drill 0.5)
  Top 0.813: v83.5,54.59 v83.5,89.52
  Bottom 0.813: R202.2 70.8,90.15 71.75,89.2 T201.3 78.74,89.52 v83.5,89.52 | JP201.1 v83.5,54.59
ERROR  (via drill 0.5)
  Top 0.61: v46.04,40.94 v46.04,26.65
  Bottom 0.61: IC101.15 v46.04,40.94 | v46.04,26.65 48.9,26.65 51.44,24.11 69.53,24.11 73.03,27.6 79.38,27.6 80.64,28.87 80.64,35.54 85.72,40.62 LED201.K
GND  (via drill 0.5)
  Top 0.406: 33.34,7.6 35.56,7.6 36.51,8.55 36.51,11.73 37.15,12.36 IC103.4 | C104.- 48.45,91.93 46.99,90.47 | R109.2 19.68,61.73 | OK101.2 22.54,50.46 23.18,49.83 C103.2
  Top 0.61: IC102.1 34.61,80.94 C101.2
  Top 0.813: 23.18,45.7 23.18,27.92 | C104.- 46.86,90.47 R107.2 41.27,84.12 40.32,83.17 IC102.1 31.75,83.17 28.26,86.66 24.77,86.66 | 24.77,86.66 V101.GND | v17.78,71.42 17.78,83.48 20.95,86.66 24.77,86.66 | 46.99,90.47 46.99,85.39 47.94,84.44 | 47.94,84.44 C105.- | 48.26,84.12 47.94,84.44 | IC101.31 51.12,53.64
  Top 1.27: 23.18,45.7 19.37,45.7 18.1,46.97 18.1,59.99 R109.2 | 20.32,27.92 18.1,30.14 | 18.1,30.14 17.14,31.09 J102.4 12.06,31.09 | 12.06,31.09 J102.3 | 18.1,30.14 18.1,27.92 | 18.1,27.92 18.1,11.09 | 18.1,11.09 J101.4 12.06,11.09 J101.5 | 18.1,27.92 20.32,27.92 | 20.32,27.92 QG101.7 23.18,27.92 23.5,27.92 IC104.9 | IC105.8 33.34,7.6 30.8,10.14 29.84,10.14 | 29.84,10.14 30.8,11.09 IC105.2 | 29.84,10.14 21.91,10.14 20.95,11.09 18.1,11.09 | 23.18,45.7 26.04,45.7 | 26.04,45.7 30.16,45.7 31.43,46.97 31.43,49.83 32.7,51.1 IC101.11 | 12.06,31.09 J102.5 | C102.2 26.04,45.7 | C103.2 23.18,45.7
  Bottom 0.813: IC101.11 34.29,51.1 36.83,53.64 IC101.31 | D101.K 6.67,83.8 8.26,82.21 8.26,78.72 15.56,71.42 v17.78,71.42
  pour Top: 99.69,99.67 43.18,99.67 43.18,79.04 50.8,79.04 50.8,0.3 99.69,0.3
KURZ
  Bottom 0.813: JP201.5 83.5,64.75 77.47,58.72 77.47,48.56 R210.2
LED-G
  Bottom 0.406: R105.1 30.8,73.01 31.43,73.64 32.7,73.64 33.02,73.96 IC101.2
LED-R
  Bottom 0.406: IC101.4 30.8,68.88 R104.1
MISO  (via drill 0.5)
  Top 0.406: v41.27,61.26 v41.27,27.29 | SV101.1 59.05,12.36 58.1,13.32 51.75,13.32 48.9,10.46 43.81,10.46 43.18,11.09 IC103.2
  Bottom 0.406: IC101.7 v41.27,61.26 | v41.27,27.29 41.91,26.65 41.91,20.62 40.64,19.35 IC104.15 40.64,15.54 43.18,13 IC103.2
MOSI  (via drill 0.5)
  Top 0.406: v39.37,63.8 v39.37,24.75 | SV101.4 56.52,6.01 55.88,5.38 52.39,5.38 50.16,7.6 v41.59,7.6
  Bottom 0.406: IC101.6 v39.37,63.8 | v39.37,24.75 39.37,20.62 38.1,19.35 IC104.14 38.1,15.54 39.37,14.27 39.37,7.85 | v41.59,7.6 39.44,7.6 39.37,7.85 | IC103.5 38.1,5.7 39.37,6.97 39.37,7.85
N$1
  Top 0.406: IC105.1 33.02,13 31.75,14.27 31.75,17.76 32.7,18.71 46.35,18.71 48.26,20.62 IC104.1
N$2
  Top 0.406: IC104.2 45.72,20.62 44.77,19.66 29.21,19.66 25.72,16.17 IC105.4
N$3  (via drill 0.5)
  Top 0.406: v23.81,50.78 28.26,50.78 OK101.3
  Bottom 0.406: R110.1 19.37,18.39 18.73,19.03 18.73,48.56 19.37,49.19 22.23,49.19 v23.81,50.78
N$4  (via drill 0.5)
  Top 0.406: R111.2 24.45,55.86 21.59,53 OK101.1 | v16.51,53 15.56,53 14.92,52.37 14.92,39.67 13.97,38.71 7.94,38.71 v7.3,38.08
  Bottom 0.406: OK101.1 v16.51,53 | v7.3,38.08 7.3,33.95 6.03,32.68 6.03,30.14 7.62,28.55 7.62,14.27 9.53,12.36 J101.3
N$5
  Top 0.813: Q201.B 55.82,57.19 60.96,52.05 OK202.3
N$6  (via drill 0.5)
  Top 0.813: v39.69,86.66 39.69,92.69 39.05,93.33 D103.C
  Bottom 0.813: C105.+ 42.86,83.48 v39.69,86.66 39.37,86.98 30.8,86.98 D102.C 28.57,87.93 27.3,86.66 V101.IN
N$7
  Top 0.813: OK201.2 58.1,89.2 59.05,88.25 59.05,77.13 59.69,76.5 68.9,76.5 70.17,75.23 D205.C
N$8
  Top 0.813: OK201.3 56.52,86.66 57.47,85.7 57.47,75.23 58.1,74.59 R208.1
N$9
  Bottom 0.61: R104.2 14.29,70.15 5.08,79.36 D101.AR
N$12
  Bottom 0.813: Q201.E 76.2,59.67 79.06,62.53 B201.-
N$13
  Bottom 0.61: R105.2 16.51,73.01 9.84,79.67 9.84,84.44 7.94,86.34 D101.AG
N$14  (via drill 0.5)
  Top 0.61: v60.01,33 55.56,33
  Top 0.813: C201.2 53.34,21.25 D204.A D203.C 54.61,29.82 55.24,30.46 55.24,33.32 | R207.1 54.29,41.57 55.24,40.62 55.24,35.86 | R206.2 55.24,35.86 | 55.24,35.86 55.24,33.32 | 55.56,33 55.24,33.32
  Bottom 0.61: v60.01,33 61.59,34.59 65.41,34.59 66.36,35.54 IC201.2
  Bottom 0.813: C201.2 59.41,20.93 L201.2
N$15
  Top 0.813: R205.1 R206.1 R204.2
  Bottom 0.813: R206.1 63.82,35.54 | R204.2 IC201.3
N$16
  Top 1.27: D202.A D201.C 66.99,12.68 70.8,16.49 TP.1
  Bottom 1.27: D201.C 71.75,14.59 79.06,14.59 91.76,27.29 X202.1
N$17
  Top 0.813: R215.1 R214.1 R213.1 63.5,55.86 OK202.4
  Bottom 0.813: R215.1 72.71,70.78 B201.+
N$18
  Top 0.813: R215.2 R214.2 R213.2 56.2,64.43 58.1,62.53 Q201.C
N$19
  Top 0.813: D203.A D204.C 63.5,18.39 62.23,17.12 60.68,17.12 L201.1
  Bottom 0.813: C201.1 59.41,18.39 L201.1 | R204.1 57.47,33 60.64,29.82 D203.A
N$20
  Top 0.813: D207.A D206.C
N$21
  Top 0.813: OK202.1 55.88,54.59 56.83,53.64 56.83,49.51 55.88,48.56 R211.1
N$22  (via drill 0.5)
  Top 0.61: v58.74,39.98 v58.74,52.05
  Bottom 0.61: v58.74,39.98 64.45,39.98 66.36,38.08 IC201.1 73.34,38.08 75.25,39.98 82.23,39.98 88.9,46.65 LED203.K | v58.74,52.05 OK202.2
N$23
  Top 0.813: D206.A R209.1 73.98,49.19 75.25,47.92 75.25,33.95 76.2,33 IC201.6
N$24
  Top 0.813: R210.1 R212.1 72.71,43.48 73.34,42.84 73.34,31.41 74.3,30.46 IC201.5
  Bottom 0.813: R210.1 C202.1
N$29
  Bottom 0.813: OK201.6 72.39,86.66 73.66,85.39 R203.2 79.38,82.85 80.33,83.8 T201.2
O'  (via drill 0.5)
  Top 1.27: D202.C D201.A 77.15,15.22 70.8,21.57 TP.2 | v89.53,66.97 v89.53,68.24 | v89.53,68.24 v89.53,17.76 v89.53,16.49 v89.53,15.22 | v89.53,68.24 v89.53,69.51
  Bottom 1.27: v89.53,17.76 v89.53,15.22 | v89.53,16.49 v89.53,15.22 | v89.53,15.22 84.14,9.82 D201.A | v89.53,66.97 v89.53,68.24 v89.53,69.51 89.53,75.86 91.12,77.45 X201.1
ONOFF  (via drill 0.5)
  Top 0.61: JP201.2 97.16,57.13 97.79,56.49 97.79,37.76 97.16,37.13 LED202.A
  Top 0.813: v82.23,57.13 82.23,89.83 75.88,96.18 68.58,96.18 67.94,95.55 R201.1
  Bottom 0.61: IC101.14 45.09,43.48 46.35,44.75 62.87,44.75 66.04,41.57 81.6,41.57 82.23,42.21 v82.23,57.13
  Bottom 0.813: OK201.7 66.04,89.2 67.94,91.1 R201.1 | JP201.2 v82.23,57.13
PLUGGED  (via drill 0.5)
  Top 0.406: v39.37,73.96 v39.37,65.07
  Bottom 0.406: R109.1 R108.2 30.48,65.07 v39.37,65.07 | IC101.39 v39.37,73.96
Q-CLK
  Top 0.406: IC101.13 33.02,46.02 30.48,43.48 30.48,27.92 | 30.48,27.92 IC104.8 | 30.48,27.92 QG101.8
ROT(FAHRSTROM)
  Top 1.27: X202.2 92.39,22.21 91.44,23.16 91.44,71.42 92.39,72.37 X201.2
SCK  (via drill 0.5)
  Top 0.406: v36.83,58.72 v36.83,26.33 | IC103.6 40.64,7.6 | IC104.13 v35.56,9.19 | v38.1,7.6 40.64,7.6 | 40.64,7.6 40.64,8.55 41.59,9.51 49.53,9.51 51.75,11.73 55.88,11.73 56.52,11.09 SV101.3
  Bottom 0.406: IC101.8 v36.83,58.72 | v36.83,26.33 36.83,20.62 35.56,19.35 IC104.13 | v35.56,9.19 37.15,7.6 v38.1,7.6
SHORT
  Bottom 0.61: IC101.17 45.4,35.86 46.67,37.13 64.77,37.13 65.09,36.81 74.93,36.81 76.2,35.54 IC201.7
SPG
  Bottom 0.61: R106.2 R107.1 41.27,78.72 43.5,76.5 IC101.40
TRACK-0-E  (via drill 0.5)
  Top 0.813: X203.1 87.95,93.01 86.04,91.1 v86.04,69.51 v86.04,3.79 v87.31,3.79 v88.58,3.79
  Bottom 0.813: v86.04,69.51 B201.AC1 76.83,69.51 73.98,66.66 67.63,66.66 66.99,66.02 R208.2 | v86.04,3.79 v87.31,3.79 v88.58,3.79 89.53,3.79 91.12,5.38 91.12,10.46 92.39,11.73 X204.1
TRACK-B-E  (via drill 0.5)
  Top 0.813: X203.2 88.9,87.93 87.31,86.34 v87.31,66.66 87.31,7.6 88.27,6.65 X204.2
  Bottom 0.813: v87.31,66.66 76.2,66.66 B201.AC2 D205.A
V-NETZTEIL  (via drill 0.5)
  Top 0.813: v14.92,90.47 22.23,90.47 24.13,92.37 D103.A | v14.92,77.45 v14.92,67.61
  Top 1.016: v84.77,91.42 v84.77,59.67
  Bottom 0.813: v14.92,90.47 v14.92,77.45 | v14.92,67.61 14.92,66.66 17.14,64.43 R108.1
  Bottom 1.016: v84.77,91.42 80.96,91.42 74.61,97.77 34.29,97.77 29.84,93.33 D103.A | v84.77,59.67 JP201.3

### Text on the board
Bottom: mbc82.brd | bottom | MBCAN-Projekt | (c) Dr.-Ing. Th. Wiesner | 01.03.2021
tNames: HW: 21.03.01 | (c) Dr.-Ing. Th. Wiesner | MBCAN-Projekt | 0 | Ring | B | 0 | B | SHORT | V+ | ON | DATA | Booster 6017 | PULS | IN | SHORT | ON | 0 | Gleis | B | OUT | 0 | Ring | B | mbc-82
